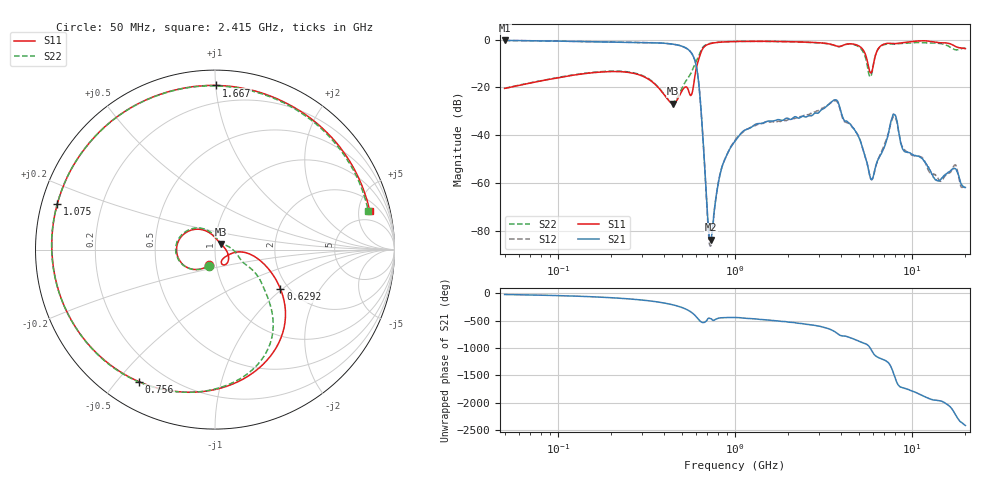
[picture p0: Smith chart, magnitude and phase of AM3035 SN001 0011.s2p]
# Hz S DB R 50
!freq MagS11 AngS11 MagS21 AngS21 MagS12 AngS12 MagS22 AngS22
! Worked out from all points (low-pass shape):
!   1601 points, 50 MHz to 20.05 GHz, reference 50 ohm
!   highest |S21| = -0.37 dB at 50 MHz (marker M1); lowest = -83.9 dB at 728.2 MHz (marker M2)
!   |S21| within 3 dB of the highest: start of sweep to 524.4 MHz
!   lowest |S11| = -26.8 dB at 447.4 MHz (marker M3), VSWR 1.10, Z = 53.3 + j3.38 ohm
!   |S11| at or under -10 dB: start of sweep to 614.9 MHz; 5.635 GHz to 6.08 GHz (445.1 MHz wide, 7.6 % of centre)
!   |S22| runs from -26.2 to -0.7 dB; largest |S21 - S12| = 0.0042
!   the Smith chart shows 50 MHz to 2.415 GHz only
!   S11 on the Smith chart (normalised r, x): 50 MHz: 0.92, -0.16; 629.2 MHz: 1.81, -0.97; 756 MHz: 0.11, -0.57; 1.075 GHz: 0.05, +0.14; 1.667 GHz: 0.09, +1.00; 2.415 GHz: 3.21, +6.58
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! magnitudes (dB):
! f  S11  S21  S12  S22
! 50 MHz  -20.5  -0.4  -0.4  -20.4
! 135.9 MHz  -14.4  -0.8  -0.8  -14.3
! 369.6 MHz  -20.1  -1.4  -1.4  -20.0
! 447.4 MHz  -26.8  -1.9  -1.9  -26.1
! 573 MHz  -22.4  -6.0  -6.1  -13.0
! 629.2 MHz  -7.4  -20.6  -20.6  -6.2
! 698.8 MHz  -2.1  -72.2  -73.7  -1.9
! 728.2 MHz  -1.7  -83.9  -86.5  -1.5
! 756 MHz  -1.4  -75.5  -75.9  -1.3
! 836.5 MHz  -1.1  -54.6  -54.4  -1.0
! 1.005 GHz  -0.8  -42.4  -41.9  -0.8
! 1.075 GHz  -0.8  -39.5  -39.6  -0.8
! 1.667 GHz  -0.8  -34.0  -34.4  -0.8
! 2.415 GHz  -1.0  -32.1  -32.0  -1.1
! 2.722 GHz  -1.2  -31.9  -31.0  -1.2
! 3.757 GHz  -2.8  -25.4  -25.9  -2.8
! 4.995 GHz  -2.6  -40.6  -40.5  -3.0
! 5.912 GHz  -13.7  -58.6  -58.7  -14.7
! 7.402 GHz  -1.6  -38.5  -38.6  -1.8
! 7.978 GHz  -1.7  -31.5  -32.3  -1.9
! 9.061 GHz  -1.3  -46.8  -46.1  -1.6
! 20.05 GHz  -3.8  -61.9  -60.9  -3.6
